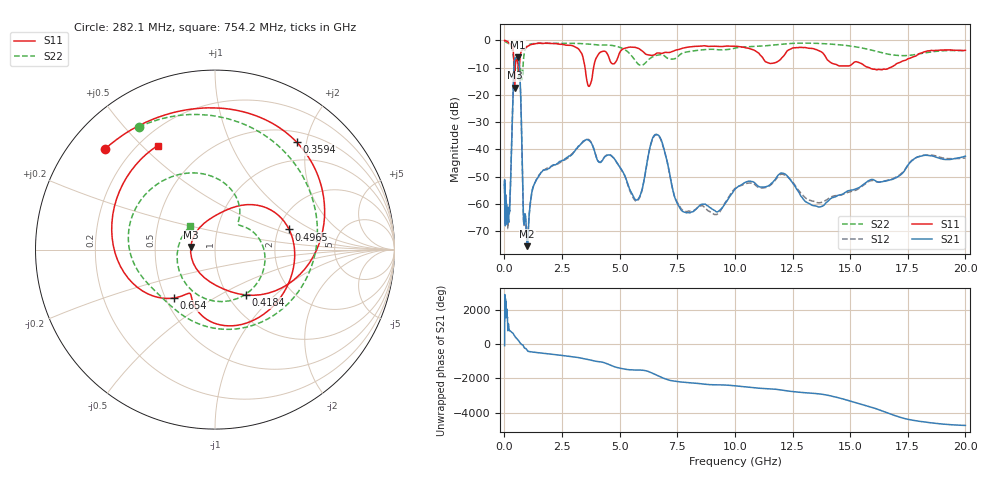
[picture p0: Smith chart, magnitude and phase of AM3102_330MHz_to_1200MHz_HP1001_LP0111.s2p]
! Date/Time: Tue, Sep 11, 2018 5:18 PM
! Network Analyzer: Agilent Technologies E8362B Rev: A.07.50.63
! Sweep from 0.010 to 20.000 GHz, 1601 Points, Sweep Type: LOG
! Power Supply: 4.949 V, 0.001 A
# Hz S DB R 50
!freq MagS11 AngS11 MagS21 AngS21 MagS12 AngS12 MagS22 AngS22
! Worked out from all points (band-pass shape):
!   1601 points, 10 MHz to 20 GHz, reference 50 ohm
!   highest |S21| = -6.25 dB at 586.3 MHz (marker M1); lowest = -75.5 dB at 988.7 MHz (marker M2)
!   |S21| within 3 dB of the highest: 417.2 MHz to 651 MHz (233.8 MHz wide, 43.8 % of centre)
!   lowest |S11| = -17.3 dB at 443 MHz (marker M3), VSWR 1.31, Z = 38.1 + j1.11 ohm
!   |S11| at or under -10 dB: 417.6 MHz to 472.2 MHz (54.67 MHz wide, 12.3 % of centre); 3.5 GHz to 3.869 GHz (369.1 MHz wide, 10 % of centre); 15.84 GHz to 16.72 GHz (881.4 MHz wide, 5.41 % of centre)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
!   |S22| runs from -14.5 to -0.2 dB; largest |S21 - S12| = 0.0089
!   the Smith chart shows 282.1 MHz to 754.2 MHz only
!   S11 on the Smith chart (normalised r, x): 282.1 MHz: 0.11, +0.39; 359.4 MHz: 0.66, +1.82; 418.4 MHz: 1.21, -0.67; 496.5 MHz: 2.29, +0.63; 654 MHz: 0.55, -0.34; 754.2 MHz: 0.27, +0.56
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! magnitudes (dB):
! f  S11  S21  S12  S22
! 10 MHz  0.0  -52.8  -53.5  -0.2
! 35.55 MHz  0.0  -62.5  -64.4  -0.4
! 126.4 MHz  -0.4  -66.2  -63.8  -0.9
! 221.4 MHz  -1.1  -62.3  -61.8  -1.3
! 282.1 MHz  -1.6  -48.1  -48.1  -1.9
! 359.4 MHz  -2.5  -23.9  -24.0  -4.3
! 418.4 MHz  -10.3  -9.1  -9.1  -7.5
! 443 MHz  -17.3  -6.8  -6.8  -8.0
! 447.2 MHz  -17.1  -6.6  -6.7  -7.9
! 496.5 MHz  -7.4  -6.5  -6.5  -6.1
! 586.3 MHz  -8.6  -6.2  -6.4  -9.8
! 654 MHz  -9.0  -9.6  -9.6  -13.1
! 754.2 MHz  -3.6  -36.2  -36.2  -14.4
! 833.3 MHz  -3.2  -66.0  -66.2  -6.6
! 988.7 MHz  -2.2  -75.5  -74.7  -2.0
! 1.59 GHz  -1.0  -48.5  -48.4  -1.0
! 3.107 GHz  -2.6  -39.8  -40.0  -1.1
! 3.617 GHz  -16.1  -36.4  -36.3  -1.3
! 5.652 GHz  -2.5  -58.2  -58.6  -7.1
! 6.58 GHz  -4.8  -34.5  -34.6  -5.5
! 7.958 GHz  -2.5  -63.2  -62.7  -4.1
! 20 GHz  -3.6  -42.5  -43.1  -3.7
